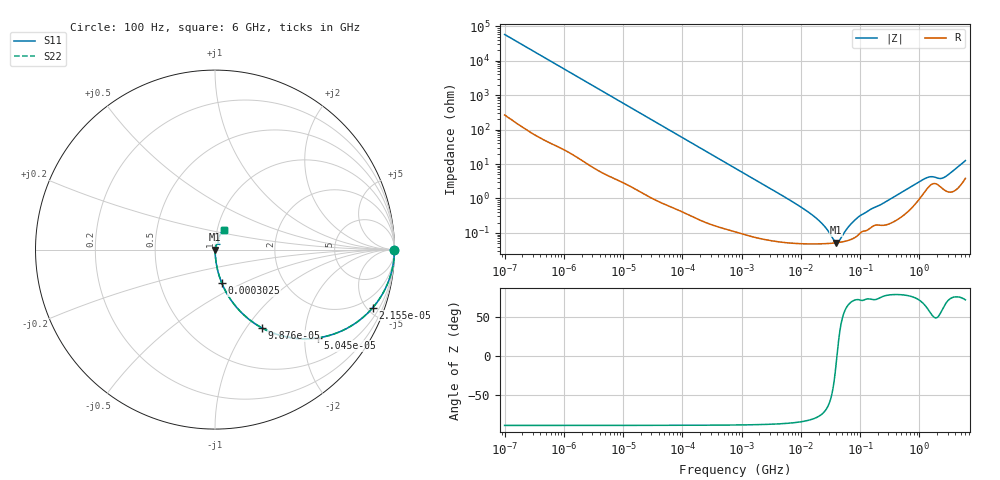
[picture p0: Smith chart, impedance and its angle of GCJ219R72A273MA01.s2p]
!Murata Part Number: GCJ219R72A273MA01
!These Parameters are Measured in Series Mode Connection
!Data Generated on Mar 13, 2026
!  o--ll--o
!Port1  Port2
!  o------o
!Operation Temp=25[degC], DC Bias Voltage=0[V]
!Freq. Start=100[Hz] Stop=6[GHz] 401[Steps]
# Hz S RI R 50
!Freq.(Hz) S11(Real) S11(Imag) S21(Real) S21(Imag) S12(Real) S12(Imag) S22(Real) S22(Imag)
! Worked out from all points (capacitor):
!   401 points, 100 Hz to 6 GHz, reference 50 ohm
!   read as one part in series: C = 27.6 nF near 109 Hz
!   lowest |Z| = 52.2 mohm at 39.84 MHz (marker M1)
!   series resonance near 40.76 MHz, so ESL is about 550 pH
!   S11 on the Smith chart (normalised r, x): 100 Hz: open; 21.55 kHz: 1.03, -5.43; 50.45 kHz: 1.01, -2.33; 98.76 kHz: 1.01, -1.19; 302.5 kHz: 1.00, -0.39; 6 GHz: 1.08, +0.24
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100  1 -0.00173  1.1e-05 0.00173  1.1e-05 0.00173  1 -0.00173
2008  0.9987 -0.0345  0.00134 0.0345  0.00134 0.0345  0.9987 -0.0345
7358  0.9838 -0.1241  0.0162 0.1241  0.0162 0.1241  0.9838 -0.1241
21550  0.8793 -0.3232  0.1207 0.3232  0.1207 0.3232  0.8793 -0.3232
40335  0.6778 -0.4646  0.3222 0.4646  0.3222 0.4646  0.6778 -0.4646
50455  0.5743 -0.4915  0.4257 0.4915  0.4257 0.4915  0.5743 -0.4915
98762  0.2632 -0.4369  0.7368 0.4369  0.7368 0.4369  0.2632 -0.4369
161617  0.1192 -0.3203  0.8808 0.3203  0.8808 0.3203  0.1192 -0.3203
302498  0.0383 -0.1874  0.9617 0.1874  0.9617 0.1874  0.0383 -0.1874
774597  0.00688 -0.076  0.9931 0.076  0.9931 0.076  0.00688 -0.076
6353432  0.000595 -0.00921  0.9994 0.00921  0.9994 0.00921  0.000595 -0.00921
1.555665e7  0.00049 -0.0033  0.9995 0.0033  0.9995 0.0033  0.00049 -0.0033
2.434276e7  0.000488 -0.00159  0.9995 0.00159  0.9995 0.00159  0.000488 -0.00159
3.64232e7  0.000509 -0.000332  0.9995 0.000332  0.9995 0.000332  0.000509 -0.000332
3.983537e7  0.000517 -6.67e-05  0.9995 6.67e-05  0.9995 6.67e-05  0.000517 -6.67e-05
4.35672e7  0.000528 0.000198  0.9995 -0.000198  0.9995 -0.000198  0.000528 0.000198
6.518806e7  0.000618 0.00145  0.9994 -0.00145  0.9994 -0.00145  0.000618 0.00145
9.326766e7  0.000875 0.00276  0.9991 -0.00276  0.9991 -0.00276  0.000875 0.00276
3.124326e8  0.00192 0.00909  0.9981 -0.00909  0.9981 -0.00909  0.00192 0.00909
1.309207e9  0.0186 0.0339  0.9814 -0.0339  0.9814 -0.0339  0.0186 0.0339
2.562649e9  0.0192 0.0343  0.9808 -0.0343  0.9808 -0.0343  0.0192 0.0343
6e9  0.0497 0.1098  0.9503 -0.1098  0.9503 -0.1098  0.0497 0.1098
